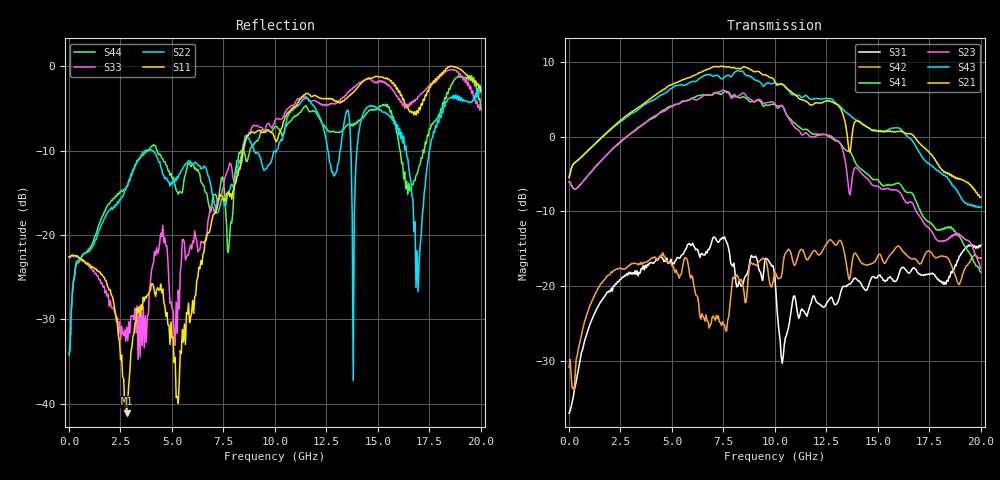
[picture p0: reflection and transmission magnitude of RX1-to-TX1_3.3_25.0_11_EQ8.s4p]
!Agilent Technologies,N5225A,MY51451112,A.09.50.13
!Agilent N5225A: A.09.50.13
!Date: Wednesday, January 31, 2018 11:04:29
!Correction: S11(Full 4 Port(1,2,3,4))
!S12(Full 4 Port(1,2,3,4))
!S13(Full 4 Port(1,2,3,4))
!S14(Full 4 Port(1,2,3,4))
!S21(Full 4 Port(1,2,3,4))
!S22(Full 4 Port(1,2,3,4))
!S23(Full 4 Port(1,2,3,4))
!S24(Full 4 Port(1,2,3,4))
!S31(Full 4 Port(1,2,3,4))
!S32(Full 4 Port(1,2,3,4))
!S33(Full 4 Port(1,2,3,4))
!S34(Full 4 Port(1,2,3,4))
!S41(Full 4 Port(1,2,3,4))
!S42(Full 4 Port(1,2,3,4))
!S43(Full 4 Port(1,2,3,4))
!S44(Full 4 Port(1,2,3,4))
!S4P File: Measurements: <S11,S12,S13,S14>,
!<S21,S22,S23,S24>,
!<S31,S32,S33,S34>,
!<S41,S42,S43,S44>:
# Hz S  RI  R 50
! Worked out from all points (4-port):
!   401 points, 10 MHz to 20 GHz, reference 50 ohm
!   strongest paths, dB at 10 MHz, 5.008 GHz, 10.01 GHz, 15 GHz, 20 GHz:
!     S21: -5.4, 7.0, 7.4, 0.8, -8.1
!     S43: -5.4, 6.5, 7.3, 0.8, -9.3
!     S23: -6.1, 4.0, 4.4, -6.6, -17.6
!     S41: -6.1, 4.1, 4.3, -5.7, -18.1
!     S42: -30.9, -17.3, -18.2, -15.9, -16.2
!     S31: -37.1, -17.3, -19.1, -18.6, -14.5
!   lowest |S11| = -41.1 dB at 2.809 GHz (marker M1), VSWR 1.02, Z = 49.7 - j0.83 ohm
!   |S11| at or under -10 dB: start of sweep to 8.446 GHz
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1e7  -0.0744 -0.00299  -0.00024 0.000545  0.0138 0.000986  0.00017 0.000387
     0.5358 0.0109  -0.0134 0.0141  -0.498 0.000593  0.0266 0.012
     0.014 0.000441  0.000168 0.000802  -0.0738 -0.004  -0.000282 0.000698
     -0.4978 0.00157  0.0259 0.012  0.5339 0.00997  -0.0133 0.0144
2.8086e9  -0.00279 -0.00834  0.0166 0.00261  0.0542 0.1085  0.018 0.000228
          1.096 -0.858  0.1954 0.00309  -0.7439 0.6795  0.1025 0.092
          0.059 0.106  0.0198 0.00317  0.0155 0.0239  0.0216 0.000392
          -0.638 0.7717  0.0912 0.0959  0.8649 -1.053  0.1874 -0.0494
7.056475e9  -0.0191 0.1319  0.0157 -0.0166  0.1356 0.0715  0.00706 -0.0323
            -2.96 0.1664  0.1146 -0.1023  1.931 -0.4418  0.0437 0.0278
            0.172 0.1258  0.0255 -0.0201  0.0289 0.1332  0.0202 -0.042
            1.567 -1.17  0.06 -0.0114  -2.177 1.346  0.1047 -0.1399
8.655675e9  -0.00956 0.3875  0.00347 -0.0085  0.0818 0.0727  -0.00769 -0.0174
            -0.9093 2.756  -0.1179 0.3732  0.2343 -1.833  -0.00911 0.13
            0.0988 0.0701  0.00925 -0.0204  0.0288 0.3879  -0.0116 -0.0292
            -0.6142 -1.682  -0.0268 0.0884  0.6066 2.508  0.1997 0.1866
1.055472e10  0.159 0.4846  -0.0265 -0.0279  0.0187 0.0262  -0.0416 -0.000231
             1.785 1.173  0.3222 0.3376  -1.355 -0.4135  0.0685 0.1864
             -0.00995 0.0454  -0.034 -0.0245  0.2241 0.4999  -0.0476 -0.0067
             -1.381 0.3321  0.0874 0.1441  2.118 -0.0527  0.4233 -0.1317
1.425288e10  0.6871 0.4249  -0.0274 0.00287  0.00232 0.0898  -0.0115 0.0124
             0.2808 -1.183  0.486 0.162  0.0218 0.5589  0.1474 0.0317
             0.0116 0.0984  -0.0129 -0.00224  0.7664 0.2757  -0.0221 0.0202
             0.4795 0.3565  0.1297 0.0551  -0.942 -0.7707  -0.1565 -0.4747
2e10  0.711 0.0676  0.023 0.0348  -0.0788 0.1626  0.0346 0.0209
      -0.00525 0.3946  0.6938 0.0751  0.0356 -0.1265  0.1541 0.0412
      -0.0794 0.1706  0.00616 0.0479  0.5639 -0.0267  0.0476 0.0205
      -0.1044 -0.0668  0.1475 0.0459  0.3159 0.128  -0.1522 -0.5323
